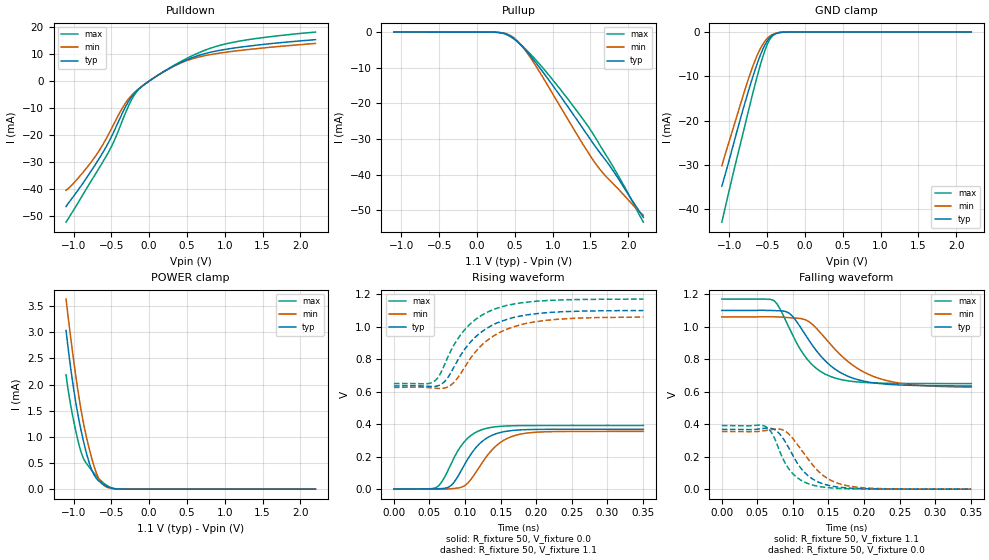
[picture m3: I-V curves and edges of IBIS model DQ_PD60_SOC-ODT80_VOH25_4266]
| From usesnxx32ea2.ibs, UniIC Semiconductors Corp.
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| DQ_PD60_SOC-ODT80_VOH25_4266
| (60 Ohm Pulldown, 80 Ohm System ODT Setting, VOH=VDDQ/2.5, 3200-4266Mbps)
[Model]   DQ_PD60_SOC-ODT80_VOH25_4266
Model_type   I/O
Vinl = 160.000mV
Vinh = 280.000mV
Vmeas = 220.000mV
Vref = 0.0mV
Cref = 0.0pF
Rref = 80.000Ohm
|   typ   min   max
|C_comp   0.834pF   0.784pF   0.884pF
C_comp_pullup   0.4170pF   0.3920pF   0.4420pF
C_comp_pulldown   0.4170pF   0.3920pF   0.4420pF
| Note: C_comp changes when the ODT circuit is enabled.
[Model Spec]
| Input threshold voltage corners
Vinl   0.1600V   0.1520V   0.1740V
Vinh   0.2800V   0.2720V   0.2940V
| Measurement voltage corners
Vmeas   0.2200V   0.2120V   0.2340V
| Timing spec test load voltage corners
Vref   0.0000V   0.0000V   0.0000V
| Dynamic Overshoot Parameters from LPDDR4 Specification
D_overshoot_ampl_h   0.30   NA   NA
D_overshoot_ampl_l   0.30   NA   NA
D_overshoot_area_h   0.1n   NA   NA
D_overshoot_area_l   0.1n   NA   NA
[Voltage Range]   1.1000V   1.0600V   1.1700V
[Pullup Reference]   1.1000V   1.0600V   1.1700V
| Junction Temperature (Ambient temp is 35C typ 95C min -40C max)
[Temperature Range]   50.0   110.0   -40.0
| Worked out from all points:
|   slope of the pulldown table from 0 to 0.165 V, typ, clamps not added: 54.7 ohm
|   slope of the pullup table from 0 to 0.165 V, typ, clamps not added: 17.7 kohm
|   GND clamp passes 1 mA (typ) near -0.45 V on its own axis
|   POWER clamp passes 1 mA (typ) near -0.88 V on its own axis
|   rising waveform, R_fixture 50, V_fixture 0.0: 20-80 % time 35ps typ, 38.6ps min, 31.9ps max; typ from 0.001 V to 0.368 V
|   falling waveform, R_fixture 50, V_fixture 1.1: 20-80 % time 53.8ps typ, 66.1ps min, 43.3ps max; typ from 1.1 V to 0.635 V
|   rising waveform, R_fixture 50, V_fixture 1.1: 20-80 % time 55.5ps typ, 58.5ps min, 51.9ps max; typ from 0.635 V to 1.1 V
|   falling waveform, R_fixture 50, V_fixture 0.0: 20-80 % time 35.1ps typ, 42.1ps min, 29.8ps max; typ from 0.368 V to 0.001 V
[Pulldown]
|   Voltage   I(typ)   I(min)   I(max)
-1.1V     -46.59mA   -40.55mA   -52.4mA
-964.7mV  -41.42mA   -36.85mA   -46.33mA
-763.4mV  -33.22mA   -29.97mA   -36.93mA
-525.8mV  -22.18mA   -19.19mA   -25.77mA
-360.8mV  -12.31mA   -10.36mA   -15.17mA
-255.2mV  -6.824mA   -6.049mA   -8.222mA
-172.7mV  -3.909mA   -3.703mA   -4.272mA
-77mV     -1.59mA    -1.563mA   -1.582mA
408.1mV   6.732mA    6.55mA     7.044mA
880mV     11.08mA    10.12mA    12.78mA
1.339V    13.02mA    11.76mA    15.45mA
2.2V      15.34mA    13.95mA    18.15mA
[GND Clamp]
|   Voltage   I(typ)   I(min)   I(max)
-1.1V     -34.75mA   -30.2mA    -42.92mA
-944.9mV  -25.23mA   -21.44mA   -31.56mA
-789.8mV  -15.73mA   -12.78mA   -20.73mA
-723.8mV  -11.94mA   -9.346mA   -16.11mA
-667.7mV  -8.911mA   -6.72mA    -12.3mA
-595.1mV  -5.401mA   -3.898mA   -7.696mA
-522.5mV  -2.665mA   -1.902mA   -3.814mA
-466.4mV  -1.3mA     -941.3uA   -1.692mA
-413.6mV  -567.7uA   -416.6uA   -621.5uA
-354.2mV  -179.6uA   -134.7uA   -160.1uA
-255.2mV  -14.6uA    -12.93uA   -8.859uA
2.2V      0A         0A         0A
[Pullup]
|   Voltage   I(typ)   I(min)   I(max)
-1.1V     4.106uA    7.431uA    1.361uA
266.2mV   -69.36uA   -66.65uA   -71.81uA
394.9mV   -631.9uA   -524.2uA   -750.4uA
507.1mV   -2.157mA   -1.952mA   -2.25mA
612.7mV   -4.374mA   -4.386mA   -4.194mA
744.7mV   -7.716mA   -8.411mA   -7.051mA
1.088V    -17.54mA   -20.45mA   -15.71mA
1.458V    -28.85mA   -33.42mA   -26.13mA
1.573V    -32.37mA   -37.08mA   -29.9mA
1.698V    -35.91mA   -40.36mA   -34.29mA
1.956V    -44.08mA   -46.07mA   -43.63mA
2.2V      -52.05mA   -51.4mA    -53.39mA
[POWER Clamp]
|   Voltage   I(typ)   I(min)   I(max)
-1.1V     3.033mA    3.633mA    2.184mA
-1.041V   2.345mA    2.929mA    1.625mA
-981.2mV  1.753mA    2.275mA    1.183mA
-911.9mV  1.2mA      1.61mA     764.5uA
-852.5mV  818.3uA    1.148mA    543.7uA
-779.9mV  447.9uA    701.4uA    396.3uA
-713.9mV  239.2uA    373uA      278.6uA
-657.8mV  146.8uA    178.9uA    190.6uA
-595.1mV  80.74uA    68.29uA    109.3uA
-486.2mV  16.78uA    10.13uA    20.96uA
-367.4mV  1.203uA    872.8nA    947.4nA
2.2V      0A         0A         0A
[Ramp]
|   typ   min   max
| 20% - 80%
dV/dt_r   220.58m/34.98p   212.91m/38.64p   234.66m/31.86p
dV/dt_f   278.79m/53.87p   259.07m/66.15p   312.07m/43.34p
| 25% - 75%
|dV/dt_r   183.82m/27.84p   177.42m/30.78p   195.55m/25.31p
|dV/dt_f   232.33m/42.89p   215.89m/52.71p   260.06m/34.44p
R_load = 50
[Rising Waveform]
R_fixture = 50
V_fixture = 0.0
|   Time   V(typ)   V(min)   V(max)
0s        727.4uV    593.5uV    534.4uV
58ps      505.6uV    12.21uV    7.106mV
67ps      2.893mV    -473.1uV   42.34mV
77ps      12.29mV    918.3uV    123.7mV
87ps      56.86mV    4.918mV    212.8mV
102ps     170.9mV    29.17mV    305.4mV
129ps     309.2mV    192.9mV    372.7mV
152ps     350.9mV    293.6mV    387.1mV
182ps     365.4mV    341.5mV    391.1mV
351ps     368.4mV    355.4mV    391.6mV
[Falling Waveform]
R_fixture   = 50
V_fixture   = 1.1
V_fixture_min = 1.06
V_fixture_max = 1.17
|   Time   V(typ)   V(min)   V(max)
0s        1.1V       1.06V      1.17V
74ps      1.099V     1.061V     1.158V
95ps      1.082V     1.055V     989.8mV
118ps     946.9mV    1.042V     811.9mV
135ps     841.8mV    981.1mV    736.6mV
154ps     756.5mV    886.2mV    691.9mV
188ps     678.2mV    751.8mV    661.3mV
224ps     649.2mV    678.1mV    652.7mV
272ps     638.3mV    641.3mV    650.3mV
351ps     635.3mV    628.2mV    649.9mV
[Rising Waveform]
R_fixture   = 50
V_fixture   = 1.1
V_fixture_min = 1.06
V_fixture_max = 1.17
|   Time   V(typ)   V(min)   V(max)
0s        635mV      626.1mV    649.8mV
55ps      631.3mV    622.3mV    659.1mV
64ps      639.5mV    619.3mV    700.4mV
77ps      694mV      631.4mV    823.7mV
88ps      779.5mV    674.8mV    913mV
105ps     891.5mV    787.2mV    1.007V
123ps     966.8mV    884.1mV    1.068V
146ps     1.024V     957.8mV    1.115V
216ps     1.086V     1.04V      1.161V
351ps     1.099V     1.059V     1.17V
[Falling Waveform]
R_fixture = 50
V_fixture = 0.0
|   Time   V(typ)   V(min)   V(max)
0s        368.5mV    355.6mV    391.7mV
58ps      374.3mV    358.9mV    391.9mV
74ps      367.4mV    370.2mV    315.1mV
87ps      307.5mV    362.6mV    178.3mV
97ps      232mV      327.4mV    109.9mV
112ps     125.4mV    240.7mV    53.84mV
129ps     59.65mV    143.3mV    24.4mV
152ps     22.03mV    58.01mV    8.687mV
183ps     6.28mV     16.71mV    2.471mV
351ps     779.8uV    697.8uV    553.4uV
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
